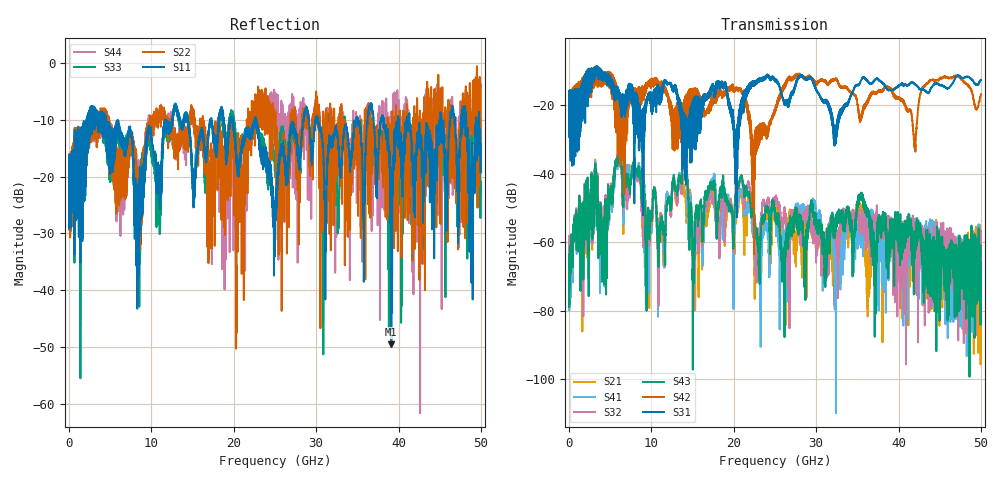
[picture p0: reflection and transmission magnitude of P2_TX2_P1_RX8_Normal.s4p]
!Keysight Technologies,N5225B,MY57041031,A.13.20.10
!Date: Friday, May 31, 2019 11:26:36
!Correction: S11(Full 4 Port(1,2,3,4))
!S12(Full 4 Port(1,2,3,4))
!S13(Full 4 Port(1,2,3,4))
!S14(Full 4 Port(1,2,3,4))
!S21(Full 4 Port(1,2,3,4))
!S22(Full 4 Port(1,2,3,4))
!S23(Full 4 Port(1,2,3,4))
!S24(Full 4 Port(1,2,3,4))
!S31(Full 4 Port(1,2,3,4))
!S32(Full 4 Port(1,2,3,4))
!S33(Full 4 Port(1,2,3,4))
!S34(Full 4 Port(1,2,3,4))
!S41(Full 4 Port(1,2,3,4))
!S42(Full 4 Port(1,2,3,4))
!S43(Full 4 Port(1,2,3,4))
!S44(Full 4 Port(1,2,3,4))
!S4P File: Measurements: <S11,S12,S13,S14>,
!<S21,S22,S23,S24>,
!<S31,S32,S33,S34>,
!<S41,S42,S43,S44>:
# Hz S  dB  R 50.0
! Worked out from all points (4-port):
!   5000 points, 10 MHz to 50 GHz, reference 50 ohm
!   strongest paths, dB at 10 MHz, 12.51 GHz, 25.01 GHz, 37.51 GHz, 50 GHz:
!     S31: -19.4, -14.8, -13.0, -12.4, -12.6
!     S42: -19.5, -24.3, -21.9, -16.0, -16.8
!     S43: -69.9, -44.9, -51.1, -60.0, -65.8
!     S32: -58.2, -46.0, -47.5, -53.3, -67.3
!     S41: -61.7, -45.0, -51.2, -70.4, -62.5
!     S21: -76.3, -45.7, -48.8, -61.4, -66.9
!   lowest |S11| = -49.5 dB at 39.13 GHz (marker M1), VSWR 1.01, Z = 50.3 + j0.0915 ohm
!   |S11| at or under -10 dB: 4.481 GHz to 11.72 GHz (7.238 GHz wide, 89.4 % of centre); 22.73 GHz to 28.43 GHz (5.702 GHz wide, 22.3 % of centre); 30.26 GHz to 34.82 GHz (4.556 GHz wide, 14 % of centre)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
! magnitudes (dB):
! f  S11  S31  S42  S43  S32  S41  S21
! 10 MHz  -19.1  -19.4  -19.5  -69.9  -58.2  -61.7  -76.3
! 6.09 GHz  -11.0  -16.4  -28.4  -34.5  -34.7  -33.7  -33.7
! 9.51 GHz  -12.9  -18.7  -13.9  -53.8  -56.0  -52.3  -54.2
! 14.01 GHz  -10.1  -31.3  -25.7  -37.1  -40.8  -38.7  -45.8
! 15.16 GHz  -24.9  -20.9  -15.5  -68.7  -69.6  -57.5  -60.1
! 39.13 GHz  -49.5  -15.6  -15.1  -53.9  -57.4  -57.5  -53.7
! 50 GHz  -14.3  -12.6  -16.8  -65.8  -67.3  -62.5  -66.9
